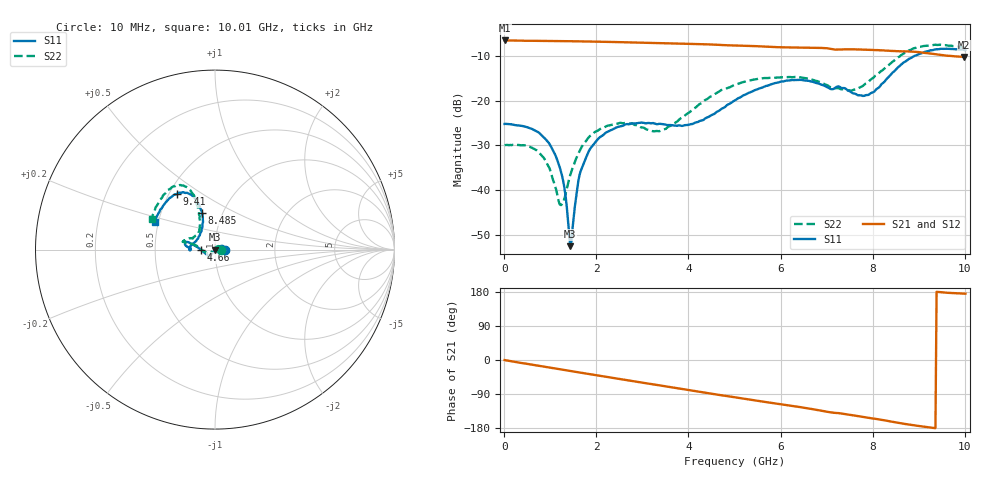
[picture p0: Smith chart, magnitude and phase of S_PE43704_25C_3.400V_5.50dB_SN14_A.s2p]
! Device ID: PE43704
! Dir: z:\PE43704\PE43704_Char_1_20130516\PE43704\AMB\3p400V\5p50dB
! Serial: 14
! Insertion: A
! Impedance: 50 ohm
! Temp: Amb
! VDD: 3.400V
! Attenuation Step: 5.50dB
! IDD: 1.140682e-01mA
#  Hz  S  RI  R  50
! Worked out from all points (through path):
!   401 points, 10 MHz to 10.01 GHz, reference 50 ohm
!   highest |S21| = -6.51 dB at 10 MHz (marker M1); lowest = -10.2 dB at 9.985 GHz (marker M2)
!   group delay of S21, straight-line fit = 52.8 ps
!   lowest |S11| = -52.5 dB at 1.435 GHz (marker M3), VSWR 1.00, Z = 50.2 - j0.125 ohm
!   |S11| at or under -10 dB: start of sweep to 8.9 GHz
!   |S22| runs from -43.3 to -7.5 dB; largest |S21 - S12| = 0.0037
!   S11 on the Smith chart (normalised r, x): 10 MHz: 1.12, +0.00; 4.66 GHz: 0.86, -0.00; 8.485 GHz: 0.80, +0.35; 9.41 GHz: 0.55, +0.39; 10.01 GHz: 0.48, +0.17
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1e7  0.055 0.000213  0.4725 -0.00185  0.4727 -0.00188  0.0318 0.000345
6.6e8  0.0419 0.0207  0.4553 -0.109  0.4553 -0.1088  0.0211 0.0196
1.01e9  0.0256 0.0177  0.437 -0.1626  0.4369 -0.1625  0.00673 0.0146
1.235e9  0.0133 0.00888  0.4214 -0.1961  0.4215 -0.196  -0.00422 0.00535
1.435e9  0.00201 -0.00125  0.4053 -0.2241  0.4053 -0.2239  -0.0137 -0.00565
1.485e9  -0.000504 -0.00374  0.4012 -0.2309  0.4012 -0.2308  -0.0157 -0.00845
1.685e9  -0.0104 -0.0142  0.3827 -0.2575  0.3827 -0.2573  -0.023 -0.0201
1.885e9  -0.0182 -0.0238  0.3624 -0.282  0.3624 -0.2819  -0.0274 -0.0304
2.235e9  -0.026 -0.0363  0.3232 -0.3211  0.3233 -0.3208  -0.0332 -0.0404
3.36e9  -0.0324 -0.0447  0.1746 -0.4061  0.175 -0.4059  -0.0378 -0.0255
4.035e9  -0.0475 -0.0265  0.076 -0.4257  0.0765 -0.4257  -0.0751 1.94e-05
4.66e9  -0.0772 -0.00185  -0.0149 -0.4217  -0.0146 -0.4216  -0.1225 0.0296
5.01e9  -0.0999 0.0146  -0.0612 -0.4103  -0.0609 -0.4107  -0.1469 0.0316
5.985e9  -0.1571 0.0431  -0.1759 -0.3557  -0.1741 -0.3564  -0.1773 0.0444
6.685e9  -0.1623 0.0215  -0.2496 -0.3021  -0.2499 -0.3017  -0.1629 0.0556
7.585e9  -0.1136 0.04  -0.3125 -0.209  -0.312 -0.2089  -0.0921 0.0956
7.96e9  -0.0828 0.0892  -0.3316 -0.1652  -0.3317 -0.1666  -0.0849 0.151
8.36e9  -0.068 0.1752  -0.3432 -0.1145  -0.3427 -0.1161  -0.0947 0.2364
8.485e9  -0.0726 0.206  -0.3465 -0.0972  -0.3451 -0.0988  -0.1042 0.2686
9.41e9  -0.2136 0.3091  -0.3294 0.00239  -0.329 0.00343  -0.2499 0.3385
9.985e9  -0.3311 0.1657  -0.3083 0.0268  -0.31 0.0278  -0.3486 0.1782
1.001e10  -0.3368 0.155  -0.309 0.0273  -0.311 0.0273  -0.3525 0.1697
